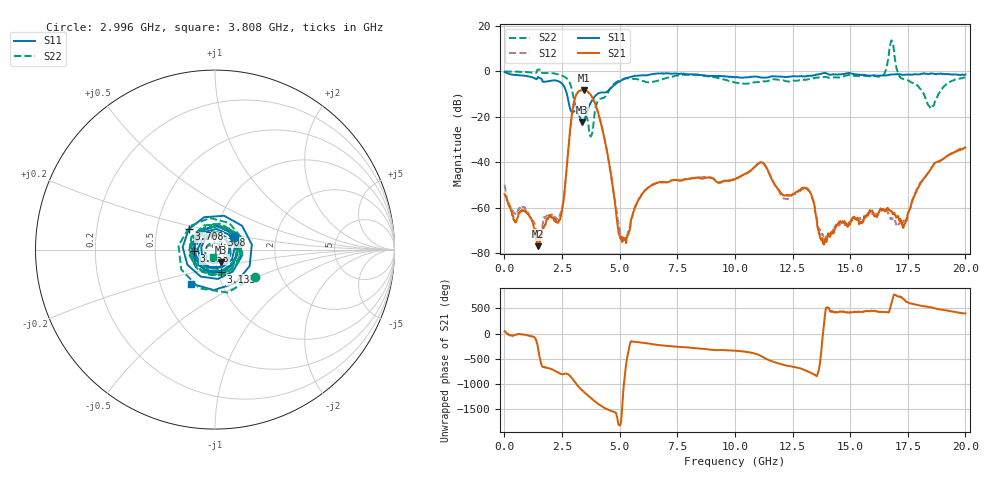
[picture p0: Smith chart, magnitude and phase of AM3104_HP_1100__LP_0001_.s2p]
!Created with skrf (http://scikit-rf.org).
# Hz S RI R 50.0
!freq ReS11 ImS11 ReS21 ImS21 ReS12 ImS12 ReS22 ImS22
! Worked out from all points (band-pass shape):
!   1601 points, 10 MHz to 20 GHz, reference 50 ohm
!   highest |S21| = -8.22 dB at 3.433 GHz (marker M1); lowest = -77.0 dB at 1.447 GHz (marker M2)
!   |S21| within 3 dB of the highest: 3.081 GHz to 3.802 GHz (720.6 MHz wide, 20.9 % of centre)
!   lowest |S11| = -22.3 dB at 3.371 GHz (marker M3), VSWR 1.17, Z = 52.7 - j7.49 ohm
!   |S11| at or under -10 dB: 2.713 GHz to 4.033 GHz (1.32 GHz wide, 39.1 % of centre)
!   |S22| runs from -28.7 to 13.6 dB; largest |S21 - S12| = 0.013
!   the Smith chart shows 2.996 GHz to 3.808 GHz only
!   S11 on the Smith chart (normalised r, x): 2.996 GHz: 1.23, +0.17; 3.133 GHz: 1.03, -0.26; 3.308 GHz: 0.94, +0.16; 3.558 GHz: 0.79, -0.02; 3.708 GHz: 0.73, +0.17; 3.808 GHz: 0.72, -0.29
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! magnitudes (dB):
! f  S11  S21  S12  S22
! 10 MHz  -0.3  -54.1  -49.8  0.0
! 1.447 GHz  -2.5  -77.0  -73.2  0.8
! 2.446 GHz  -4.9  -64.0  -62.0  -1.7
! 2.996 GHz  -17.9  -14.6  -14.6  -11.4
! 3.133 GHz  -17.8  -10.0  -10.0  -16.7
! 3.308 GHz  -21.2  -8.4  -8.5  -16.6
! 3.346 GHz  -22.0  -8.3  -8.3  -16.6
! 3.371 GHz  -22.3  -8.2  -8.3  -16.7
! 3.433 GHz  -22.2  -8.2  -8.2  -17.5
! 3.558 GHz  -18.6  -8.6  -8.7  -19.7
! 3.708 GHz  -14.6  -9.8  -9.9  -27.9
! 3.808 GHz  -12.7  -11.3  -11.3  -27.3
! 5.057 GHz  -4.1  -73.8  -72.1  -3.9
! 6.682 GHz  -0.9  -49.0  -49.1  -4.1
! 10.01 GHz  -2.6  -47.6  -47.5  -4.9
! 11.17 GHz  -2.8  -40.1  -40.3  -4.6
! 13.34 GHz  -2.0  -55.2  -55.3  -3.2
! 13.87 GHz  -0.7  -76.3  -72.9  -2.5
! 16.68 GHz  -1.5  -61.2  -62.8  7.1
! 17.34 GHz  -1.6  -67.7  -66.4  -3.5
! 18.48 GHz  -0.9  -43.4  -43.6  -16.3
! 20 GHz  -1.4  -33.6  -33.5  -2.7
